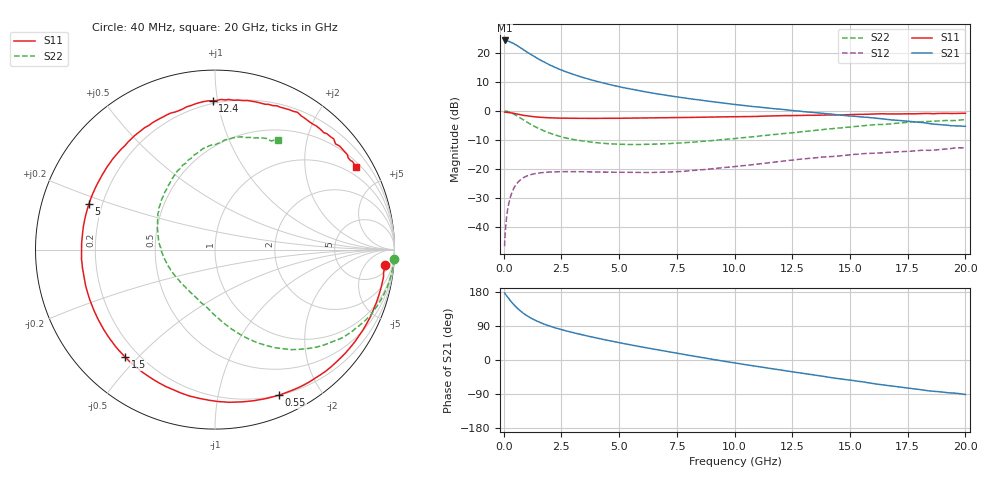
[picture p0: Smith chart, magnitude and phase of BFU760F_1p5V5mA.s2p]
! Filename:  P:\Prog\Test\Noise\ATS_data\Testdata_Net\Split files Spar\BFU760F_2W_C1_Bias1_1.5V_5mA_60mA_D.s2p
! Date/Time: Mon 06/Feb/2012 15:06:35
! BFU760_2W_C1_Bias1_1.5V_5mA_60mA_R.s2p
! MDIF S-parameter v. bias file
! BFU760_2W_C1_1.5V_5mA_60mA
! Date/time Fri Mar 18 11:09:37 2011
! bias mode 1
! bias variable = I_out
! VAR bias_var= 1
! VAR V_out= 1.5001
! VAR I_out= 5.0100
! VAR V_in= 0.7578
! VAR I_in= 0.0140
! Device data file deembeded for feedlines and parallel
! Original file: \Split files Spar\BFU760_2W_C1_Bias1_1.5V_5mA_60mA_R.s2p
! Feed-files: PR003V01_101208_Feed1.s2p, PR003V01_101208_Feed2.s2p
! Parallel-file: PR003V01_101208_Par.s2p
# MHz S MA R 50
!  Freq-MHz  S11-mag  S11-arg  S21-mag  S21-arg  S12-mag  S12-arg  S22-mag  S22-arg
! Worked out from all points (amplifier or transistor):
!   167 points, 40 MHz to 20 GHz, reference 50 ohm
!   highest |S21| = 24.2 dB at 50 MHz (marker M1)
!   |S21| within 3 dB of that: start of sweep to 822.2 MHz
!   unconditionally stable (mu >= 1): 6.07 GHz to 13.14 GHz
!   at 550 MHz: K = 0.07, MSG = 23.9 dB, |S12| = -25.2 dB
!   at 4.2 GHz: K = 0.68, MSG = 15.4 dB, |S12| = -21.1 dB
!   at 20 GHz: K = 0.80, MSG = 3.7 dB, |S12| = -12.7 dB
!   S11 on the Smith chart (normalised r, x): 40 MHz: 9, -17; 550 MHz: 0.20, -1.52; 1.5 GHz: 0.15, -0.46; 5 GHz: 0.15, +0.17; 12.4 GHz: 0.18, +0.97; 20 GHz: 0.66, +3.55
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40  0.9519 -5.3  16.29 176.8  0.004692 86.9  0.9976 -3.1
50  0.949 -7.1  16.31 175.5  0.006336 88.0  0.9964 -3.9
60  0.9477 -7.6  16.09 174.8  0.007213 84.9  0.9968 -4.6
80  0.9501 -10.5  16.23 173.3  0.009452 84.5  0.9948 -6.2
140  0.9463 -18.2  16.04 168.3  0.01647 80.3  0.986 -10.8
280  0.9301 -35.9  15.37 157.2  0.03183 70.8  0.9477 -21.2
420  0.9076 -52.4  14.54 147.3  0.04496 61.9  0.8909 -30.6
550  0.8866 -66.2  13.57 139.1  0.05475 54.6  0.8289 -38.4
750  0.8544 -84.7  12.08 128.2  0.06626 45.3  0.7401 -48.4
1000  0.8215 -103.2  10.37 117.2  0.07564 36.4  0.6428 -58.4
1250  0.7971 -118.0  8.967 108.4  0.08146 29.7  0.5637 -66.1
1500  0.7806 -129.8  7.85 101.1  0.08497 24.5  0.5011 -72.6
1850  0.7649 -142.9  6.611 92.5  0.08787 18.9  0.4355 -80.2
2250  0.7532 -154.4  5.56 84.5  0.08952 14.3  0.3827 -87.4
3400  0.7444 -177.6  3.796 66.5  0.08979 6.1  0.305 -104.9
5000  0.7467 160.1  2.611 45.8  0.08755 1.9  0.266 -127.9
6800  0.7584 140.6  1.921 25.4  0.08783 2.5  0.2701 -153.2
10200  0.7977 109.4  1.266 -9.6  0.112 3.8  0.3411 160.0
12400  0.8285 90.8  1.029 -30.2  0.141 -2.2  0.4159 133.6
13400  0.8385 83.0  0.9395 -39.1  0.1549 -7.6  0.456 122.3
16800  0.8864 55.7  0.6997 -68.5  0.1942 -27.7  0.5981 86.6
20000  0.9106 30.5  0.5424 -91.1  0.2316 -50.3  0.7053 59.9
